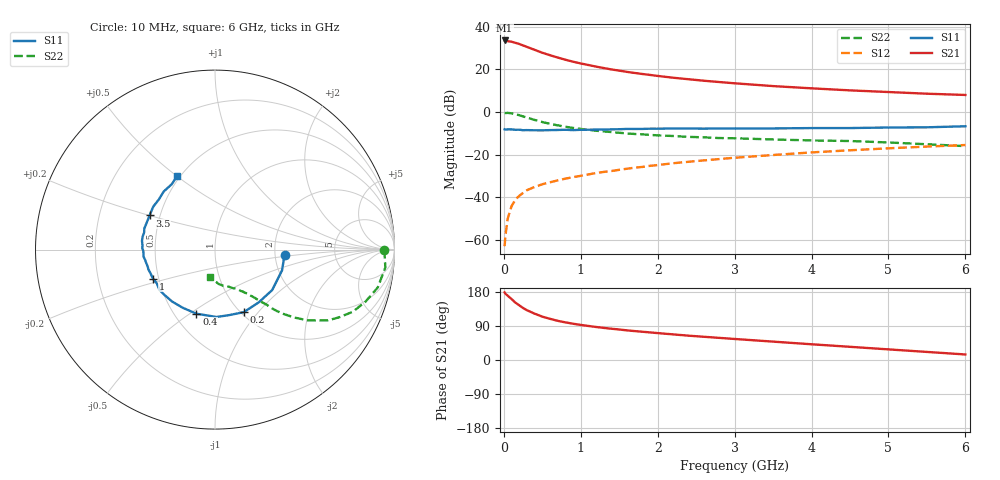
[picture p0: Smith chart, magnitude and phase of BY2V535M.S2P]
! SIEMENS Small Signal Semiconductors
! BFY420
! Si NPN RF SIEGET Grounded Emitter Transistor in MICRO-X
! VCE = 2.5 V  IC = 35 mA
! Common Emitter S-Parameters:  October  1996
# GHz  S  MA  R  50
!  f  S11  S21  S12  S22
! GHz  MAG  ANG  MAG  ANG  MAG  ANG  MAG  ANG
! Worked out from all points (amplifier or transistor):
!   36 points, 10 MHz to 6 GHz, reference 50 ohm
!   highest |S21| = 33.7 dB at 10 MHz (marker M1)
!   |S21| within 3 dB of that: start of sweep to 298 MHz
!   unconditionally stable (mu >= 1): start of sweep to 14.22 MHz; 1.509 GHz to end of sweep
!   at 250 MHz: K = 0.39, MSG = 34.7 dB, |S12| = -38.1 dB
!   at 1.4 GHz: K = 0.99, MSG = 23.9 dB, |S12| = -27.7 dB
!   at 6 GHz: K = 1.06, MAG = 10.3 dB, |S12| = -15.5 dB
!   S11 on the Smith chart (normalised r, x): 10 MHz: 2.28, -0.15; 200 MHz: 1.03, -0.84; 400 MHz: 0.64, -0.53; 1 GHz: 0.47, -0.18; 3.5 GHz: 0.44, +0.20; 6 GHz: 0.48, +0.50
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0.01  0.3922 -4.2  48.15 178.3  0.0007 117.7  0.9402 -0.1
0.02  0.3872 -7.7  47.94 175.0  0.0012 93.9  0.9452 -1.5
0.1  0.3903 -35.3  45 160.9  0.0061 78.1  0.931 -13.1
0.15  0.3818 -50.5  42.37 151.5  0.0087 74.4  0.8873 -19.1
0.2  0.3835 -65.4  39.79 144.4  0.0107 71.6  0.8421 -24.3
0.25  0.3735 -77.7  36.76 137.2  0.0125 67.6  0.7879 -28.6
0.3  0.3756 -88.6  33.98 131.4  0.0145 65.8  0.7411 -32.2
0.4  0.3718 -106.1  29 122.3  0.0173 64.0  0.6511 -37.3
0.5  0.3707 -119.1  24.75 114.4  0.02 63.2  0.5814 -40.6
0.6  0.3753 -129.6  21.66 108.7  0.0222 62.6  0.5278 -43.0
0.7  0.3779 -137.7  19.1 103.4  0.0246 62.8  0.4856 -44.8
0.8  0.3826 -144.1  16.95 99.3  0.0271 61.9  0.4501 -46.1
1  0.3815 -154.9  13.85 92.6  0.0316 63.7  0.4003 -47.8
1.1  0.3828 -159.6  12.72 89.8  0.0341 63.2  0.3807 -49.1
1.4  0.3908 -169.3  10.01 82.5  0.041 64.0  0.3377 -51.2
1.6  0.4001 -174.5  8.784 78.2  0.0463 63.5  0.3132 -53.0
2.2  0.4097 173.2  6.403 67.6  0.0624 61.0  0.2726 -57.9
2.8  0.4111 163.3  5.067 58.4  0.0782 57.5  0.2442 -62.5
3.5  0.4111 152.4  4.07 48.5  0.0975 52.5  0.2258 -68.0
4.5  0.4195 138.3  3.227 34.8  0.1259 44.1  0.2077 -76.8
5.5  0.437 123.4  2.694 21.3  0.154 34.5  0.1744 -90.3
6  0.4621 117.0  2.517 14.6  0.1673 29.6  0.1576 -99.5
